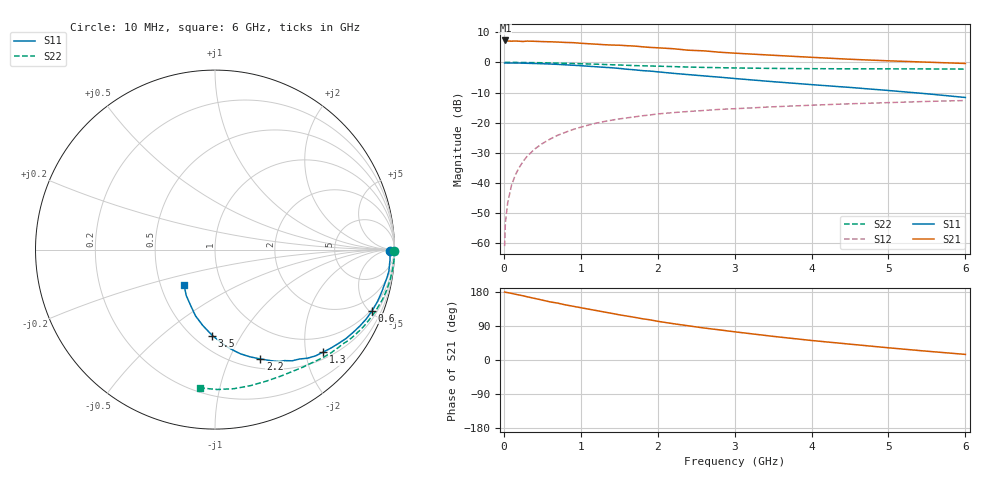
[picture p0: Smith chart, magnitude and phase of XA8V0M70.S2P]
! SIEMENS Discrete & RF Semiconductors
! BFY180
! Si NPN RF Bipolar Junction Transistor in MICRO-X
! VCE = 8 V  IC = 0.7 mA
! Common Emitter S-Parameters:  May  1997
# GHz  S  MA  R  50
!  f  S11  S21  S12  S22
! GHz  MAG  ANG  MAG  ANG  MAG  ANG  MAG  ANG
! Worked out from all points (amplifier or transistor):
!   36 points, 10 MHz to 6 GHz, reference 50 ohm
!   highest |S21| = 7.3 dB at 20 MHz (marker M1)
!   |S21| within 3 dB of that: start of sweep to 2.305 GHz
!   unconditionally stable (mu >= 1): 5.323 GHz to end of sweep
!   at 250 MHz: K = 0.05, MSG = 19.9 dB, |S12| = -32.8 dB
!   at 1.4 GHz: K = 0.41, MSG = 12.5 dB, |S12| = -19.2 dB
!   at 6 GHz: K = 1.02, MAG = 5.2 dB, |S12| = -12.6 dB
!   S11 on the Smith chart (normalised r, x): 10 MHz: 80, -17; 600 MHz: 0.89, -5.19; 1.3 GHz: 0.64, -2.35; 2.2 GHz: 0.61, -1.31; 3.5 GHz: 0.61, -0.76; 6 GHz: 0.66, -0.28
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0.01  0.9763 -0.3  2.253 179.3  0.0009 79.9  0.9984 -0.3
0.02  0.9784 -0.6  2.31 178.7  0.0022 91.6  0.9999 -0.5
0.05  0.9753 -1.5  2.26 177.8  0.0047 85.1  0.9989 -1.2
0.1  0.9767 -3.6  2.249 175.8  0.0092 89.4  0.9991 -2.4
0.15  0.9759 -5.6  2.26 173.6  0.0137 86.2  0.9987 -3.6
0.2  0.9762 -7.1  2.245 171.4  0.0181 85.9  0.9961 -4.8
0.3  0.9669 -10.5  2.254 166.9  0.0275 81.9  0.9938 -7.2
0.4  0.9585 -14.2  2.237 162.6  0.0366 79.6  0.991 -9.5
0.6  0.9397 -21.2  2.196 153.4  0.0535 74.0  0.9802 -14.1
0.9  0.8965 -31.1  2.124 141.8  0.0773 66.5  0.9586 -20.9
1.1  0.864 -37.3  2.038 134.3  0.0914 61.6  0.9415 -25.0
1.3  0.8295 -43.6  1.967 126.8  0.1045 57.3  0.9241 -29.1
1.5  0.7947 -49.6  1.926 119.3  0.1156 53.2  0.906 -32.9
1.7  0.7536 -55.3  1.865 112.6  0.1252 49.5  0.8846 -36.5
2.2  0.6595 -67.5  1.685 95.9  0.1472 41.3  0.8516 -44.8
2.6  0.5974 -76.3  1.554 84.5  0.1596 36.2  0.8261 -50.5
3  0.5408 -83.6  1.423 74.4  0.1707 31.4  0.8086 -56.0
3.5  0.4789 -91.8  1.313 62.4  0.1837 26.5  0.7947 -62.4
4  0.428 -99.2  1.214 51.5  0.1951 21.8  0.7867 -68.8
4.5  0.3847 -106.4  1.127 41.8  0.2062 17.3  0.7832 -75.5
5.5  0.3018 -122.1  1.009 23.2  0.2254 8.9  0.7796 -89.1
6  0.2621 -131.0  0.96 14.8  0.2334 4.3  0.7749 -96.0
